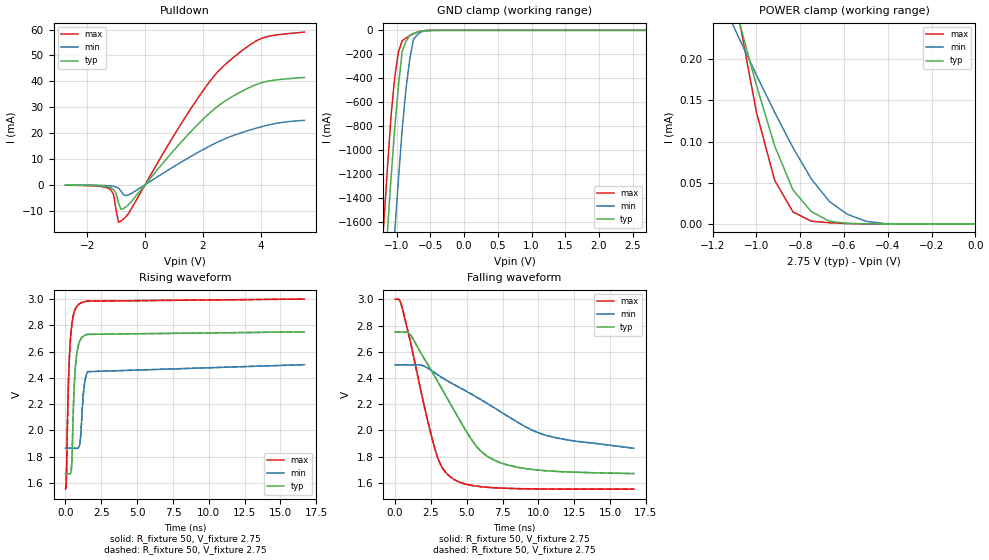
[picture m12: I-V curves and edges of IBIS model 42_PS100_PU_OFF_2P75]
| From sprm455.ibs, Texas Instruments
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|   Model Cell 42_PS100_PU_OFF_2P75
|IDG09_OUM42_PS100_PU_OFF_2P75
[Model]   42_PS100_PU_OFF_2P75
Model_type   I/O_open_drain
Polarity   Non-Inverting
Enable   Active-Low
Vinl =  0.7V
Vinh =  1.7V
Cref =  15pF
Rref =  100.00M
Vref =  0V
Vmeas =  1.375
C_comp   4.287p   4.203p   4.656p
[Model Spec]
Vinl   0.7V   0.7V   0.7V
Vinh   1.7V   1.7V   1.7V
[Temperature Range]   25   125   -40
[Voltage Range]   2.75   2.5   3
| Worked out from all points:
|   slope of the pulldown table from 0 to 0.412 V, typ, clamps not added: 73.2 ohm
|   GND clamp passes 1 mA (typ) near -0.51 V on its own axis
|   POWER clamp passes 1 mA (typ) near -1.78 V on its own axis
|   rising waveform, R_fixture 50, V_fixture 2.75: 20-80 % time 256ps typ, 272ps min, 257ps max; typ from 1.67 V to 2.75 V
|   rising waveform, R_fixture 50, V_fixture 2.75: 20-80 % time 256ps typ, 272ps min, 257ps max; typ from 1.67 V to 2.75 V
|   falling waveform, R_fixture 50, V_fixture 2.75: 20-80 % time 3.51ns typ, 6.06ns min, 1.83ns max; typ from 2.75 V to 1.67 V
|   falling waveform, R_fixture 50, V_fixture 2.75: 20-80 % time 3.51ns typ, 6.06ns min, 1.83ns max; typ from 2.75 V to 1.67 V
| Nom Voltages:
|   VDD=1.1, VDDS=2.75, VSS=0, VSSS=0
| Min Voltages:
|   VDD=1, VDDS=2.5, VSS=0, VSSS=0
| Max Voltages:
|   VDD=1.2, VDDS=3, VSS=0, VSSS=0
[POWER_clamp]
|   voltage   I(typ)   I(min)   I(max)
-2.75V    2.078mA    1.233mA    3.105mA
-1.111V   278.5uA    243.6uA    297.9uA
-1.083V   250uA      227.7uA    254.3uA
-1.056V   222.8uA    212uA      214.7uA
-1V       168.4uA    180.8uA    135.5uA
-916.7mV  94.71uA    135.4uA    52.81uA
-833.3mV  41.32uA    92.62uA    14.65uA
-750mV    15.05uA    54.86uA    3.347uA
-666.7mV  3.185uA    27.16uA    1.455uA
-583.3mV  666.6nA    11.53uA    482.3nA
-416.7mV  18.12nA    529.1nA    5.125nA
0V        77.76pA    12.31nA    1.013pA
[Pulldown]
|   voltage   I(typ)   I(min)   I(max)
-2.75V    -158.8uA   -86.66uA   -198.2uA
-1.25V    -956.2uA   -405.1uA   -1.484mA
-1.083V   -1.925mA   -649.1uA   -4.056mA
-1V       -3.428mA   -904uA     -10mA
-916.7mV  -7.154mA   -1.402mA   -14.51mA
-833.3mV  -9.533mA   -2.46mA    -14.08mA
-666.7mV  -8.643mA   -4.227mA   -12.48mA
-500mV    -6.859mA   -3.549mA   -9.807mA
1.333V    17.54mA    9.305mA    25.13mA
2.583V    30.97mA    16.88mA    44.51mA
4V        39.37mA    22.37mA    56.5mA
5.5V      41.47mA    24.89mA    59.04mA
[GND_clamp]
|   voltage   I(typ)   I(min)   I(max)
-2.75V    -17.22A    -18.08A    -16.72A
-1.194V   -2.2A      -3.135A    -1.654A
-1.139V   -1.714A    -2.64A     -1.18A
-1.083V   -1.24A     -2.152A    -725.2mA
-1.028V   -818.3mA   -1.688A    -392.4mA
-972.2mV  -463.1mA   -1.245A    -179.9mA
-916.7mV  -174.9mA   -824.1mA   -87.46mA
-861.1mV  -92.21mA   -492.7mA   -64.95mA
-805.6mV  -42.31mA   -243.6mA   -45.13mA
-750mV    -25.22mA   -76.56mA   -27.99mA
-472.2mV  -309.9uA   -1.019mA   -105.7uA
2.694V    76.04pA    15.31nA    740.1fA
[Ramp]
| variable   typ   min   max
dV/dt_f 0.64882601/3.5189394n 0.38228636/6.0684802n 0.87054957/1.8323815n
dV/dt_r 13.940975m/0.1000467n 10.778284m/0.16658179n 15.388667m/67.143474p
R_load = 50
[Rising Waveform]
R_fixture = 50
V_fixture = 2.75
V_fixture_min = 2.5
V_fixture_max = 3
|   time   V(typ)   V(min)   V(max)
0s        1.67V      1.864V     1.551V
67.41ps   1.67V      1.864V     1.647V
218.1ps   1.669V     1.864V     2.398V
351.8ps   1.672V     1.864V     2.7V
444.9ps   1.767V     1.863V     2.806V
664.6ps   2.437V     1.863V     2.918V
932.9ps   2.661V     1.871V     2.96V
1.29ns    2.72V      2.322V     2.978V
1.54ns    2.731V     2.447V     2.984V
16.67ns   2.75V      2.5V       3V
[Rising Waveform]
R_fixture = 50
V_fixture = 2.75
V_fixture_min = 2.5
V_fixture_max = 3
|   time   V(typ)   V(min)   V(max)
0s        1.67V      1.864V     1.551V
67.41ps   1.67V      1.864V     1.647V
218.1ps   1.669V     1.864V     2.398V
351.8ps   1.672V     1.864V     2.7V
444.9ps   1.767V     1.863V     2.806V
664.6ps   2.437V     1.863V     2.918V
932.9ps   2.661V     1.871V     2.96V
1.29ns    2.72V      2.322V     2.978V
1.54ns    2.731V     2.447V     2.984V
16.67ns   2.75V      2.5V       3V
[Falling Waveform]
R_fixture = 50
V_fixture = 2.75
V_fixture_min = 2.5
V_fixture_max = 3
|   time   V(typ)   V(min)   V(max)
0s        2.75V      2.5V       3V
493.6ps   2.751V     2.5V       2.938V
1.107ns   2.724V     2.5V       2.659V
2.115ns   2.533V     2.485V     2.15V
2.892ns   2.389V     2.431V     1.819V
3.906ns   2.194V     2.362V     1.641V
5.786ns   1.864V     2.248V     1.573V
7.416ns   1.751V     2.138V     1.559V
10.65ns   1.691V     1.959V     1.552V
16.67ns   1.67V      1.864V     1.551V
[Falling Waveform]
R_fixture = 50
V_fixture = 2.75
V_fixture_min = 2.5
V_fixture_max = 3
|   time   V(typ)   V(min)   V(max)
0s        2.75V      2.5V       3V
493.6ps   2.751V     2.5V       2.938V
1.107ns   2.724V     2.5V       2.659V
2.115ns   2.533V     2.485V     2.15V
2.892ns   2.389V     2.431V     1.819V
3.906ns   2.194V     2.362V     1.641V
5.786ns   1.864V     2.248V     1.573V
7.416ns   1.751V     2.138V     1.559V
10.65ns   1.691V     1.959V     1.552V
16.67ns   1.67V      1.864V     1.551V
